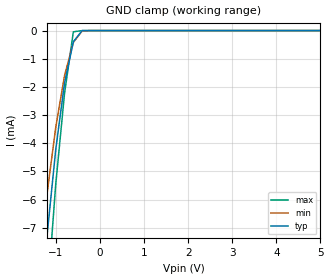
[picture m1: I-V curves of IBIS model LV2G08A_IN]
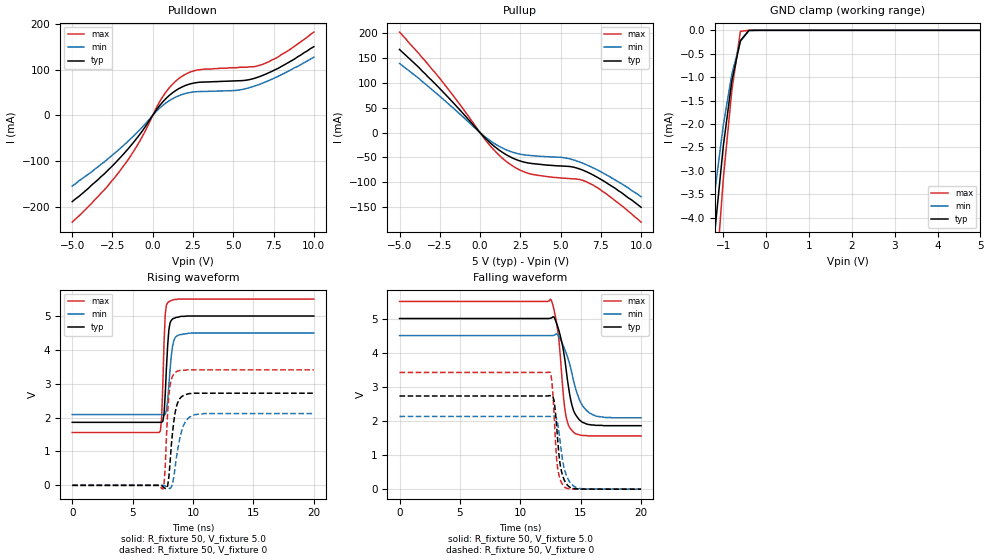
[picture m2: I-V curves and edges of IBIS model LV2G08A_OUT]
|/_/_/_/_/_/_/_/_/_/_/_/_/_/_/_/_/_/_/_/_/_/_/_/_/_/_/_/_/_/_/_/_/_/_/_/_/_/
|   Renesas Electronics Corp.
|   Multi Purpose Semiconductor Digital IC Design Group
|   IBIS Model of HD74LV2G08A
|   5.0V Dual 2-input AND Gates,  SSOP-8(8pin) Package
|   History
|   V1.0   April   1, 2003   : First release.
|/_/_/_/_/_/_/_/_/_/_/_/_/_/_/_/_/_/_/_/_/_/_/_/_/_/_/_/_/_/_/_/_/_/_/_/_/_/
[IBIS Ver]   2.1
[Comment Char]  |_char
[File name]   l2g08s5.ibs
[File Rev]   1.1
[Date]   April 1, 2003
[Source]   Data created from SPICE simulations at
|   Renesas Electronics Corp.
[Notes]   RLC value of the Package is determined by assuming typical
|   conditions.
[Disclaimer]   This information is for modeling purposes only, and is not
|   guaranteed.
[Copyright]   Copyright 2003, Renesas Electronics Corp.,
|   All Rights Reserved.
|   Component  HD74LV2G08A
[Component]   HD74LV2G08A
[Manufacturer]  Renesas Electronics Corp.
[Package]
|   typ   min   max
R_pkg   0.099   0.095   0.102
L_pkg   1.740nH   1.680nH   1.790nH
C_pkg   0.140pF   0.140pF   0.150pF
[Pin]   signal_name   model_name   R_pin   L_pin   C_pin
1   1A   LV2G08A_IN   0.102   1.780nH   0.140pF
2   1B   LV2G08A_IN   0.097   1.710nH   0.150pF
3   2Y   LV2G08A_OUT   0.095   1.680nH   0.150pF
4   GND   GND   0.102   1.790nH   0.140pF
5   2A   LV2G08A_IN   0.101   1.790nH   0.140pF
6   2B   LV2G08A_IN   0.097   1.710nH   0.150pF
7   1Y   LV2G08A_OUT   0.097   1.710nH   0.150pF
8   VCC   POWER   0.102   1.790nH   0.140pF
| Models and submodels in the file (2): LV2G08A_IN (Input), LV2G08A_OUT (Output)
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|   Model  LV2G08A_IN
[Model]   LV2G08A_IN
Model_type  Input
Vinl = 1.50V
Vinh = 3.50V
| variable   typ   min   max
C_comp   2.35pF   2.25pF   2.45pF
| variable   typ   min   max
[Temperature range]   25   85   -40
| variable   typ   min   max
[Voltage range]   5.0V   4.5V   5.5V
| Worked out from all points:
|   GND clamp passes 1 mA (typ) near -0.68 V on its own axis
[GND Clamp]
|   Voltage   I(typ)   I(min)   I(max)
-5V       -128mA     -106mA     -157mA
-1.4V     -11mA      -8.74mA    -14.7mA
-1.2V     -7.33mA    -5.84mA    -9.68mA
-1V       -4.23mA    -3.44mA    -5.46mA
-800mV    -1.86mA    -1.6mA     -2.23mA
-600mV    -396uA     -418uA     -43uA
-400mV    -474nA     -10.9uA    -2.94nA
5V        10.1pA     35.9pA     10pA
|   Model  LV2G08A_OUT
[Model]   LV2G08A_OUT
Model_type  Output
Polarity   Inverting
Vmeas = 2.5V
| variable   typ   min   max
C_comp   6.85pF   6.75pF   6.95pF
| variable   typ   min   max
[Temperature range]   25   85   -40
| variable   typ   min   max
[Voltage range]   5.0V   4.5V   5.5V
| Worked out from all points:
|   slope of the pulldown table from 0 to 0.75 V, typ, clamps not added: 22 ohm
|   slope of the pullup table from 0 to 0.75 V, typ, clamps not added: 31.4 ohm
|   GND clamp passes 1 mA (typ) near -0.78 V on its own axis
|   rising waveform, R_fixture 50, V_fixture 5.0: 20-80 % time 289ps typ, 356ps min, 224ps max; typ from 1.86 V to 5 V
|   rising waveform, R_fixture 50, V_fixture 0: 20-80 % time 467ps typ, 665ps min, 310ps max; typ from 0 V to 2.72 V
|   falling waveform, R_fixture 50, V_fixture 5.0: 20-80 % time 867ps typ, 1.2ns min, 615ps max; typ from 5 V to 1.86 V
|   falling waveform, R_fixture 50, V_fixture 0: 20-80 % time 469ps typ, 608ps min, 363ps max; typ from 2.73 V to 0 V
[Pullup]
|   Voltage   I(typ)   I(min)   I(max)
-5V       167mA      139mA      202mA
-2.4V     85.2mA     70.3mA     105mA
200mV     -6.98mA    -5.55mA    -8.94mA
1V        -30.6mA    -24.1mA    -39.5mA
1.6V      -43.9mA    -34.1mA    -57.2mA
2.4V      -56.1mA    -42.7mA    -74mA
3.2V      -62mA      -46.2mA    -83.6mA
5.2V      -67.4mA    -50.4mA    -91.6mA
5.8V      -69.4mA    -54.8mA    -92.9mA
6.6V      -78.5mA    -64.5mA    -98.7mA
7.8V      -99.8mA    -84mA      -122mA
10V       -150mA     -129mA     -180mA
[Pulldown]
|   Voltage   I(typ)   I(min)   I(max)
-5V       -189mA     -155mA     -234mA
-3V       -128mA     -102mA     -163mA
-1.6V     -76.4mA    -59.1mA    -101mA
-800mV    -41.6mA    -31.5mA    -56.3mA
600mV     28.4mA     20.9mA     39.7mA
1V        42.6mA     31.4mA     59.1mA
1.6V      57.9mA     42.5mA     79.9mA
2.8V      71.9mA     51.8mA     99.3mA
5.2V      75.3mA     54.5mA     104mA
6.8V      86.9mA     70mA       111mA
8.4V      115mA      96.1mA     141mA
10V       150mA      127mA      182mA
[GND Clamp]
|   Voltage   I(typ)   I(min)   I(max)
-5V       -76.6mA    -64mA      -93.9mA
-1.4V     -6.55mA    -5.21mA    -8.67mA
-1.2V     -4.33mA    -3.47mA    -5.69mA
-1V       -2.48mA    -2.03mA    -3.18mA
-800mV    -1.08mA    -936uA     -1.28mA
-600mV    -219uA     -237uA     -20.5uA
-400mV    -248nA     -6.13uA    -1.4nA
5V        5.14pA     37.3pA     5pA
[Ramp]
| variable   typ   min   max
dV/dt_r   1.636/469.2p   1.276/668.6p   2.049/311.9p
dV/dt_f   1.882/863.0p   1.447/1.200n   2.363/614.7p
R_load = 50ohms
[Rising Waveform]
R_fixture = 50
V_fixture = 5.0
V_fixture_min = 4.5
V_fixture_max = 5.5
C_fixture = 0p
|   Time   V(typ)   V(min)   V(max)
0s        1.86V      2.09V      1.56V
7.2ns     1.86V      2.09V      1.56V
7.4ns     1.86V      2.09V      1.98V
7.6ns     2.11V      2.07V      4.2V
7.7ns     2.7V       2.1V       5.05V
8ns       4.59V      2.96V      5.42V
8.2ns     4.87V      3.81V      5.46V
8.5ns     4.94V      4.35V      5.49V
9.2ns     4.99V      4.47V      5.5V
20ns      5V         4.5V       5.5V
[Rising Waveform]
R_fixture = 50
V_fixture = 0
C_fixture = 0p
|   Time   V(typ)   V(min)   V(max)
0s        373pV      814nV      68pV
7.5ns     -33.9mV    4.13mV     -113mV
7.7ns     -95.4mV    -20.8mV    553mV
7.9ns     -9.59mV    -65.5mV    2.17V
8.1ns     677mV      -92.6mV    2.96V
8.4ns     1.86V      228mV      3.28V
8.7ns     2.41V      990mV      3.37V
9.2ns     2.65V      1.76V      3.4V
10.1ns    2.72V      2.08V      3.41V
20ns      2.72V      2.12V      3.41V
[Falling Waveform]
R_fixture = 50
V_fixture = 5.0
V_fixture_min = 4.5
V_fixture_max = 5.5
C_fixture = 0p
|   Time   V(typ)   V(min)   V(max)
0s        5V         4.5V       5.5V
12.5ns    5.01V      4.5V       5.57V
13ns      4.86V      4.55V      4.88V
13.3ns    4.51V      4.4V       3.96V
13.7ns    3.77V      4.08V      2.31V
14.1ns    2.75V      3.65V      1.8V
14.4ns    2.31V      3.19V      1.67V
14.9ns    2.03V      2.62V      1.59V
15.7ns    1.89V      2.24V      1.56V
20ns      1.86V      2.09V      1.56V
[Falling Waveform]
R_fixture = 50
V_fixture = 0
C_fixture = 0p
|   Time   V(typ)   V(min)   V(max)
0s        2.73V      2.13V      3.42V
12.5ns    2.74V      2.13V      3.42V
12.6ns    2.74V      2.14V      3.2V
12.8ns    2.59V      2.14V      2.18V
13ns      1.88V      2.07V      904mV
13.1ns    1.42V      1.92V      593mV
13.3ns    724mV      1.39V      287mV
13.6ns    300mV      667mV      86.7mV
14.8ns    6.88mV     28.3mV     1.34mV
20ns      -27.5uV    -61.5uV    -8.48uV
